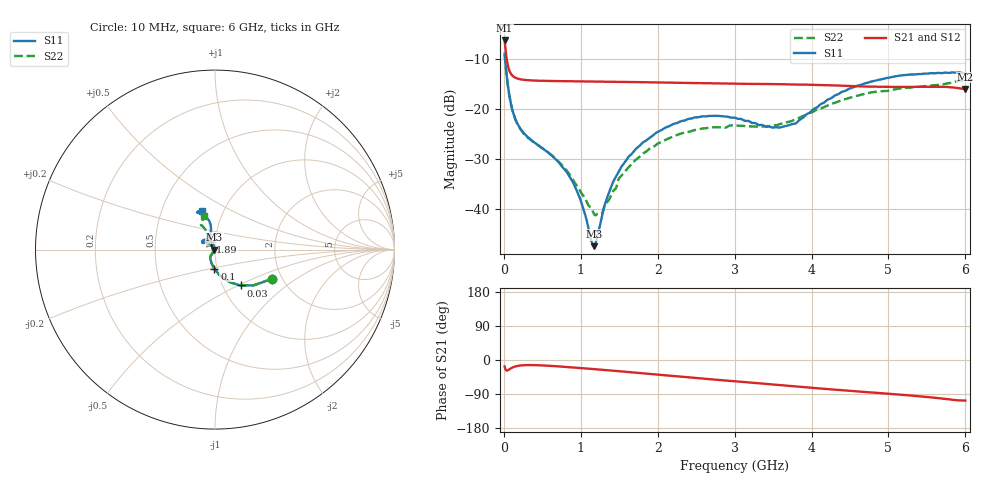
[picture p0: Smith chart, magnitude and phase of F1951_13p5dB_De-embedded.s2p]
! Integrated Device Technology
! Corporate Headquarters
! 6024 Silver Creek Valley Road
! San Jose, CA 95138  USA
! Phone:  1-408-284-8200
! Toll Free:  1-800-223-1366
! Webpage:  http://www.idt.com/
! Timing and RF Division
! 515 Groton Road, Suite 102
! Westford, MA 01886-6024
! Device:  F1951
! Description: 6-bit 0.5 dB Digital Step Attenuator
! Frequency:  100.0 -  4000.00 MHz
! Package:  4x4 mm Thin QFN Plastic Package: 24 pin
! Ports:  2 RF, 6 DC
!  Pin  1  = NC
!  Pin  2  = RF1  =  Port 1
!  Pin  3  = GND
!  Pin  4  = NC
!  Pin  5  = Serial Data Out (SDO)
!  Pin  6  = NC
!  Pin  7  = Reset Bar ( RSTb)
!  Pin  8  = Clock (CLK)
!  Pin  9  = Chip Select Bar (CSb)
!  Pin 10  = NC
!  Pin 11  = Serial Data In (SDI)
!  Pin 12  = NC
!  Pin 13  = NC
!  Pin 14  = VDD
!  Pin 15  = NC
!  Pin 16  = GND
!  Pin 17  = RF2  =  Port 2
!  Pin 18  = NC
!  Pin 19  = GND
!  Pin 20  = GND
!  Pin 21  = GND
!  Pin 22  = GND
!  Pin 23  = GND
!  Pin 24  = GND
! State:  27
! Atten State:  13.5 dB
! Voltage:  +3.30 Volts
! Current:  0.486 mA
! Data:  The device was measured on a F195X evaluation board which has
!  individual transmission lines to the RF pins.  Data was collected
!  de-embedded using a Automatic Fixture Removal [AFR] (Keysight Technologies).
!  The reference plane is the edge of the package pin.
! Misc:  Lot Code  1225BCA
!  Action Tracker AT0399
! Date Measured:  2018-09-13
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# GHz S dB R 50
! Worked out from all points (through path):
!   600 points, 10 MHz to 6 GHz, reference 50 ohm
!   highest |S21| = -6.25 dB at 10 MHz (marker M1); lowest = -16.0 dB at 6 GHz (marker M2)
!   group delay of S21, straight-line fit = 45.7 ps
!   lowest |S11| = -47.4 dB at 1.17 GHz (marker M3), VSWR 1.01, Z = 49.6 + j0.0407 ohm
!   |S11| at or under -10 dB: 16.35 MHz to end of sweep
!   |S22| runs from -41.3 to -9.0 dB; largest |S21 - S12| = 0.00037
!   S11 on the Smith chart (normalised r, x): 10 MHz: 1.78, -0.66; 30 MHz: 1.21, -0.51; 100 MHz: 0.97, -0.21; 1.89 GHz: 0.95, +0.09; 6 GHz: 0.80, +0.36
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0.01  -8.90 -26.8  -6.25 -17.2  -6.26 -17.2  -8.97 -27.1
0.03  -12.21 -54.5  -9.13 -27.4  -9.13 -27.5  -12.30 -54.8
0.06  -16.08 -76.1  -11.72 -26.3  -11.72 -26.3  -16.20 -76.6
0.1  -19.47 -91.6  -13.09 -21.1  -13.09 -21.1  -19.56 -92.3
0.17  -22.69 -106.8  -13.84 -16.1  -13.84 -16.1  -22.83 -107.4
0.26  -24.79 -116.5  -14.13 -13.8  -14.13 -13.7  -24.98 -117.7
0.72  -30.75 -120.7  -14.39 -17.0  -14.39 -17.1  -30.64 -126.8
0.89  -34.40 -119.6  -14.44 -19.6  -14.44 -19.6  -33.92 -127.8
1.01  -38.79 -122.6  -14.47 -21.5  -14.47 -21.5  -36.86 -131.7
1.17  -47.43 174.5  -14.49 -24.0  -14.49 -24.0  -40.92 -160.1
1.27  -41.79 118.4  -14.50 -25.7  -14.50 -25.7  -40.95 166.5
1.44  -33.99 108.4  -14.54 -28.7  -14.54 -28.7  -36.12 136.5
1.6  -30.00 109.6  -14.56 -31.4  -14.57 -31.4  -32.01 128.2
1.89  -25.81 118.3  -14.63 -36.6  -14.63 -36.6  -27.96 130.3
2.01  -24.48 122.8  -14.66 -38.8  -14.66 -38.8  -26.82 133.2
2.49  -21.64 138.8  -14.78 -47.3  -14.78 -47.3  -24.17 143.9
3.01  -21.74 151.0  -14.92 -56.3  -14.92 -56.2  -23.23 149.0
3.59  -23.67 129.3  -15.00 -66.3  -15.01 -66.3  -22.98 130.5
4.01  -20.22 103.6  -15.13 -73.5  -15.13 -73.5  -20.59 117.5
4.49  -15.90 101.1  -15.36 -81.5  -15.36 -81.4  -17.75 116.2
5.01  -13.70 110.3  -15.55 -89.1  -15.55 -89.1  -16.31 119.4
6  -12.84 107.8  -15.97 -107.1  -15.97 -107.1  -14.01 107.5
